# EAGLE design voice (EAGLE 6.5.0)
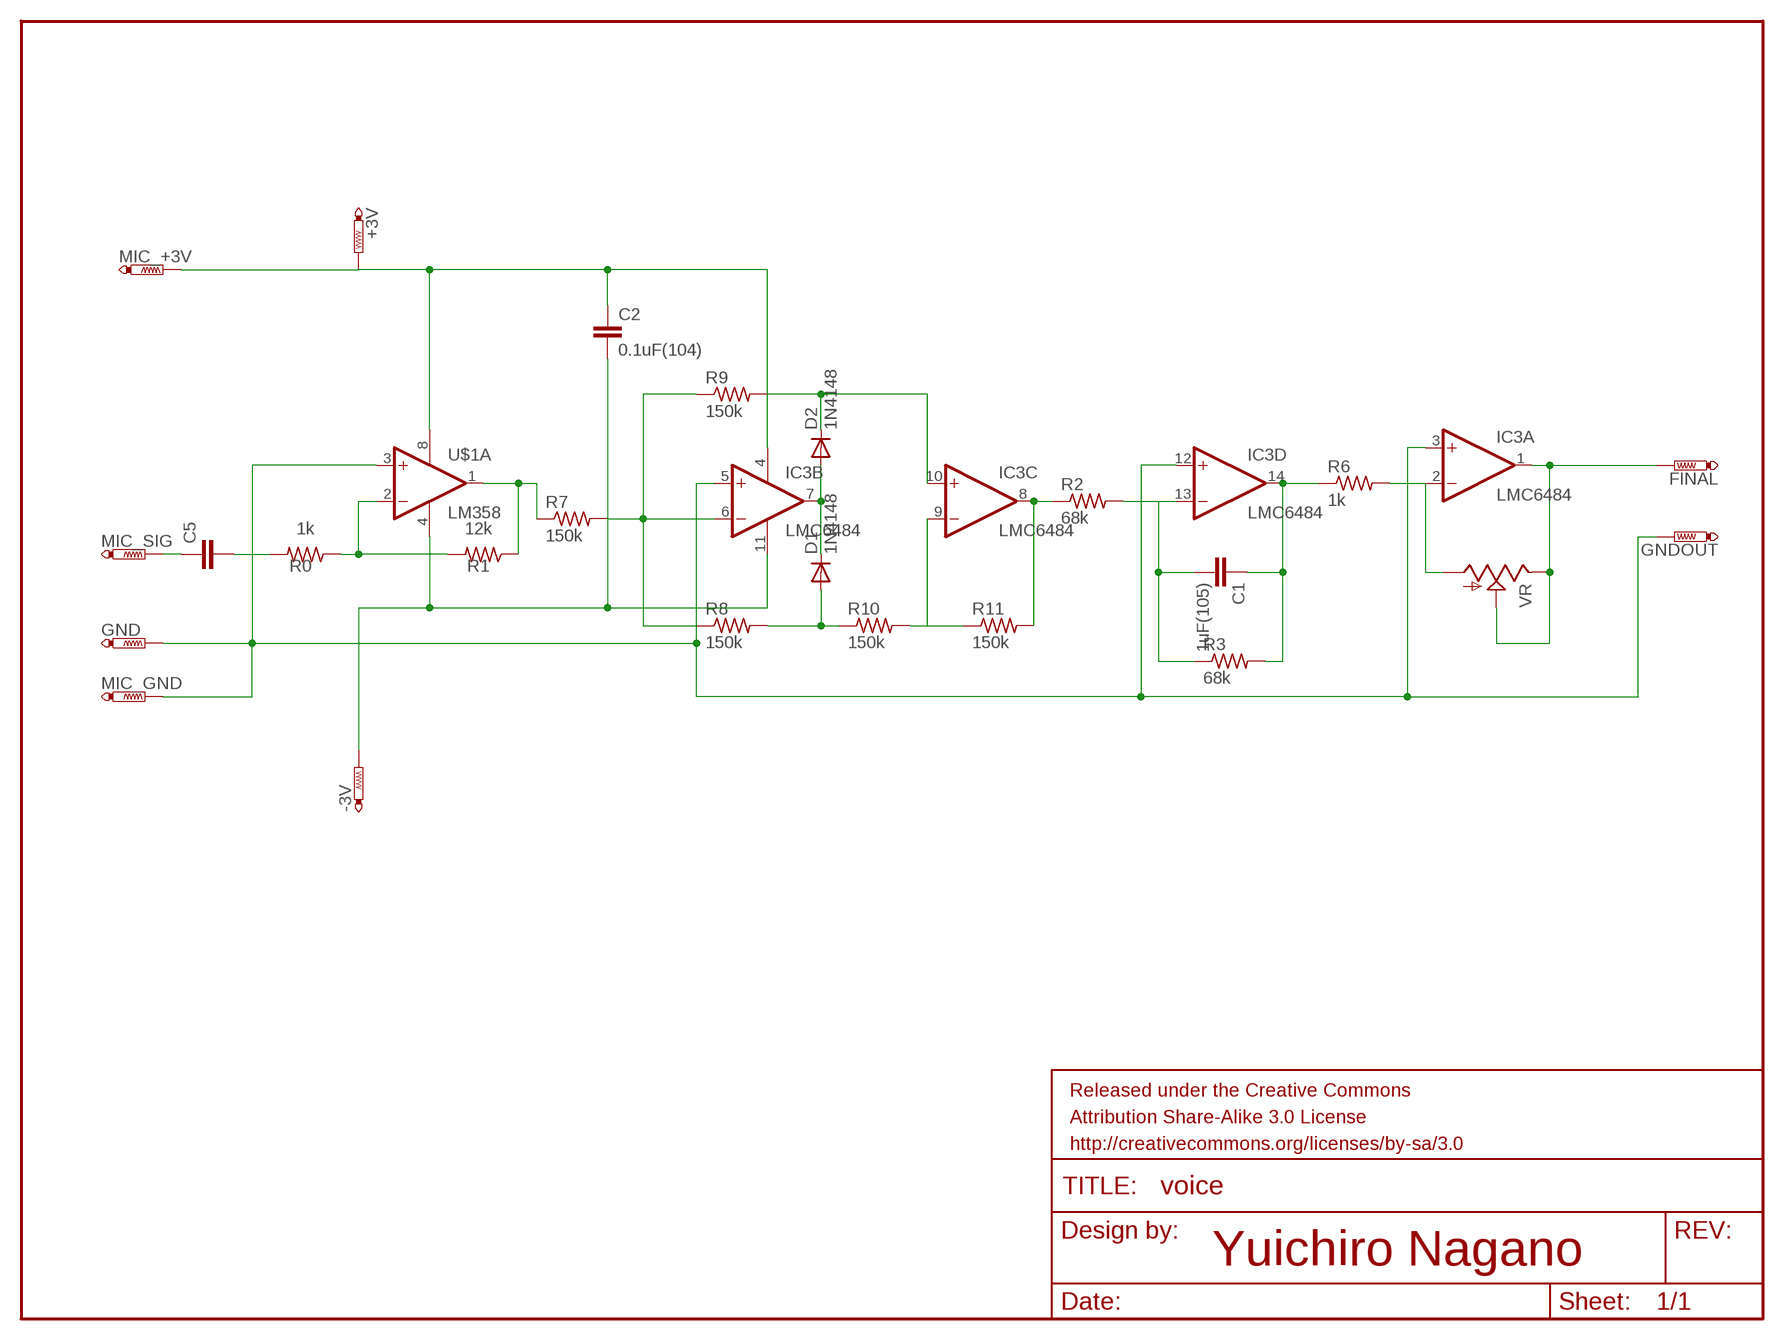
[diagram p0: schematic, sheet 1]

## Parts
+3V  PTR1PAD1-13Y  [P1-13Y]
-3V  PTR1PAD1-13Y  [P1-13Y]
C1  1uF(105)  C2,5-3  [C2.5-3]
C2  0.1uF(104)  C2,5-3  [C2.5-3]
C5  C5/5  [C5B5]
D1  1N4148  1N4148DO35-7  [DO35-7]
D2  1N4148  1N4148DO35-7  [DO35-7]
FINAL  PTR1PAD1-13Y  [P1-13Y]
FRAME1  FRAME-LETTER  [CREATIVE_COMMONS]
GND  PTR1PAD1-13Y  [P1-13Y]
GNDOUT  PTR1PAD1-13Y  [P1-13Y]
IC3  LMC6484  LM324N  [DIL14]
MIC_+3V  PTR1PAD1-13Y  [P1-13Y]
MIC_GND  PTR1PAD1-13Y  [P1-13Y]
MIC_SIG  PTR1PAD1-13Y  [P1-13Y]
R0  1k  R-US_0204/2V  [0204V]
R1  12k  R-US_0204/2V  [0204V]
R2  68k  R-US_0204/2V  [0204V]
R3  68k  R-US_0204/2V  [0204V]
R6  1k  R-US_0204/2V  [0204V]
R7  150k  R-US_0204/2V  [0204V]
R8  150k  R-US_0204/2V  [0204V]
R9  150k  R-US_0204/2V  [0204V]
R10  150k  R-US_0204/2V  [0204V]
R11  150k  R-US_0204/2V  [0204V]
U$1  LM358  [DIL8]
VR  TRIM_US-B25P  [B25P]

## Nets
N$1: IC3.9(C:-IN) R10.2 R11.1
N$2: D1.C D2.A IC3.7(B:OUT)
N$3: -3V.TP C2.2 IC3.11(P:V-) U$1.4(P:V-)
N$4: R1.1 R7.1 U$1.1(A:OUT)
N$5: R0.1 R1.2 U$1.2(A:-IN)
N$6: C5.1 MIC_SIG.TP
N$7: D1.A R8.2 R10.1
N$8: +3V.TP C2.1 IC3.4(P:V+) MIC_+3V.TP U$1.8(P:V+)
N$9: C5.2 R0.2
N$10: IC3.8(C:OUT) R2.1 R11.2
N$12: GND.TP GNDOUT.TP IC3.3(A:+IN) IC3.5(B:+IN) IC3.12(D:+IN) MIC_GND.TP U$1.3(A:+IN)
N$15: IC3.6(B:-IN) R7.2 R8.1 R9.1
N$16: D2.C IC3.10(C:+IN) R9.2
N$17: C1.2 IC3.13(D:-IN) R2.2 R3.1
N$18: C1.1 IC3.14(D:OUT) R3.2 R6.1
N$19: IC3.2(A:-IN) R6.2 VR.A
N$21: FINAL.TP IC3.1(A:OUT) VR.E VR.S
Unconnected: U$1.5(B:+IN) U$1.6(B:-IN) U$1.7(B:OUT)

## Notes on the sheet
- Yuichiro Nagano

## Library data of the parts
+3V -3V FINAL GND GNDOUT MIC_+3V MIC_GND MIC_SIG = testpad:PTR1: TEST PIN
C1 C2 C5 = capacitor-wima:C: CAPACITOR
D1 D2 = diode:1N4148: DIODE
FRAME1 = SparkFun-Aesthetics:FRAME-LETTER: Schematic Frame
IC3 = linear:LM324: OP AMP
R0 R1-R3 R6-R11 = resistor:R-US_: RESISTOR, American symbol
U$1 = atari:LM358: Dual General Purpose, Rail-to-Rail Output Operational Amplifier
VR = pot:TRIM_US-: POTENTIOMETER

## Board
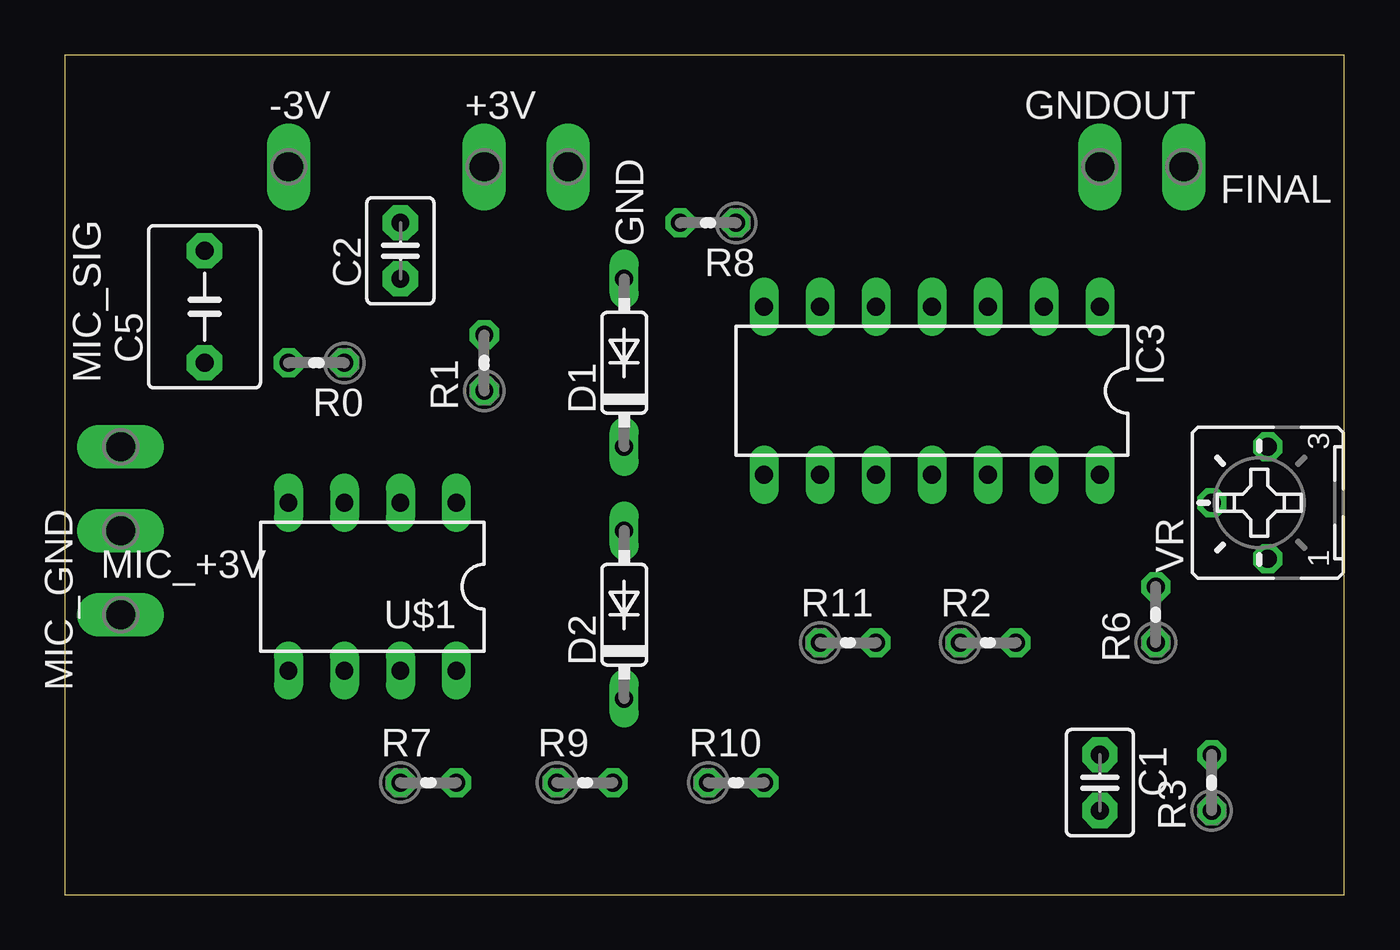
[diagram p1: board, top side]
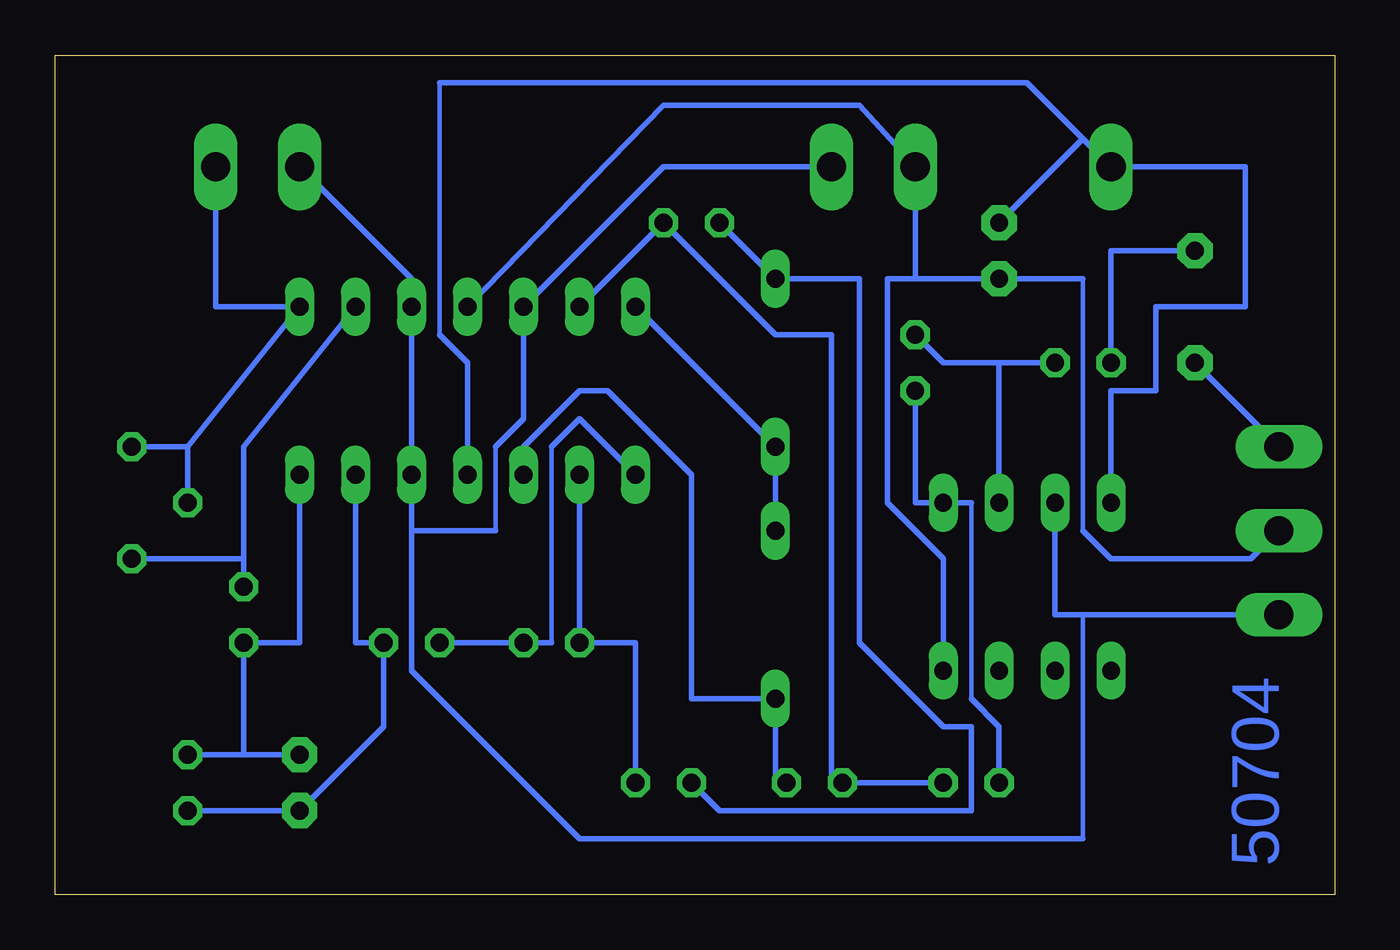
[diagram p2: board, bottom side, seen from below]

Size 58.09 x 38.09 mm. Coordinates in mm from the lower left corner, seen from the top.
Outline: 0,0 58.09,0 58.09,38.09 0,38.09 0,0
Copper layers (1*16): Top 0.035mm / dielectric 1.5mm / Bottom 0.035mm
Design rules "default": minimum track width 10mil, minimum drill 24mil, track to track 8mil, track to pad 8mil, pad to pad 8mil, via to via 8mil, smd to smd 8mil, copper to edge 40mil, drill to drill 8mil, minimum pad ring 10mil, minimum via ring 8mil, stop-mask expansion 4mil, vias tented up to drill 0mil, thermal gap 10mil

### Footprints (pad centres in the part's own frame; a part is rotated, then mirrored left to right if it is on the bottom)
P1-13Y = drill 1.321 pad 1.905 long: TP 0,0
C2.5-3 = drill 0.813 pad 1.6 octagon: 1 -1.27,0; 2 1.27,0
C5B5 = drill 0.813 pad 1.6 octagon: 1 -2.54,0; 2 2.54,0
DO35-7 = drill 0.813 long: A 3.81,0; C -3.81,0
DIL14 = drill 0.813 long: 1 -7.62,-3.81; 2 -5.08,-3.81; 3 -2.54,-3.81; 4 0,-3.81; 5 2.54,-3.81; 6 5.08,-3.81; 7 7.62,-3.81; 8 7.62,3.81; 9 5.08,3.81; 10 2.54,3.81; 11 0,3.81; 12 -2.54,3.81; 13 -5.08,3.81; 14 -7.62,3.81
0204V = drill 0.813 octagon: 1 -1.27,0; 2 1.27,0
DIL8 = drill 0.813 long: 1 -3.81,-3.81; 2 -1.27,-3.81; 3 1.27,-3.81; 4 3.81,-3.81; 5 3.81,3.81; 6 1.27,3.81; 7 -1.27,3.81; 8 -3.81,3.81
B25P = drill 0.813 octagon: A -2.54,0; E 2.54,0; S 0,2.54

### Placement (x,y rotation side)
+3V  19.05,33.02 0 top
-3V  10.16,33.02 0 top
C1  46.99,5.08 270 top
C2  15.24,29.21 90 top
C5  6.35,26.67 90 top
D1  25.4,24.13 90 top
D2  25.4,12.7 90 top
FINAL  50.8,33.02 0 top
FRAME1  not placed on the board
GND  22.86,33.02 180 top
GNDOUT  46.99,33.02 0 top
IC3  39.37,22.86 180 top
MIC_+3V  2.54,16.51 90 top
MIC_GND  2.54,12.7 90 top
MIC_SIG  2.54,20.32 90 top
R0  11.43,24.13 180 top
R1  19.05,24.13 90 top
R2  41.91,11.43 0 top
R3  52.07,5.08 90 top
R6  49.53,12.7 90 top
R7  16.51,5.08 0 top
R8  29.21,30.48 180 top
R9  23.62,5.08 0 top
R10  30.48,5.08 0 top
R11  35.56,11.43 0 top
U$1  13.97,13.97 180 top
VR  54.61,17.78 90 top

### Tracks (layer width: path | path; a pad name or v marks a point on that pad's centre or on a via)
N$1
  Bottom 0.254: R10.2 31.75,11.43 R11.1 IC3.9
N$2
  Bottom 0.254: D2.A D1.C IC3.7
N$3
  Bottom 0.203: 40.64,36.83 40.64,25.4
  Bottom 0.254: U$1.4 10.16,22.86 8.13,22.86 8.13,26.67 4.06,26.67 4.06,33.02 -3V.TP 11.43,34.29 | IC3.11 39.37,24.13 40.64,25.4 | 40.64,36.83 13.97,36.83 11.43,34.29 | 11.43,34.29 C2.2
N$4
  Bottom 0.203: 16.51,17.78 16.51,8.89
  Bottom 0.254: R7.1 15.24,7.62 16.51,8.89 | 16.51,17.78 U$1.1 19.05,17.78 R1.1
N$5
  Bottom 0.254: 15.24,24.13 U$1.2 | R0.1 15.24,24.13 | R1.2 17.78,24.13 15.24,24.13
N$6
  Bottom 0.254: MIC_SIG.TP C5.1
N$7
  Bottom 0.254: R8.2 D1.A 21.59,27.94 21.59,11.43 17.78,7.62 16.51,7.62 16.51,3.81 27.94,3.81 R10.1
N$8
  Bottom 0.203: 11.43,27.94 11.43,16.51
  Bottom 0.254: IC3.4 30.48,35.81 21.59,35.81 +3V.TP 19.05,27.94 | U$1.8 17.78,15.24 20.32,17.78 20.32,27.94 19.05,27.94 | 19.05,27.94 C2.1 11.43,27.94 | MIC_+3V.TP 3.81,15.24 10.16,15.24 11.43,16.51
N$9
  Bottom 0.254: R0.2 10.16,29.21 C5.2
N$10
  Bottom 0.203: 35.56,11.43 35.56,20.32
  Bottom 0.254: R2.1 R11.2 35.56,11.43 | IC3.8 34.29,21.59 35.56,20.32
N$12
  Bottom 0.203: 11.43,2.54 11.43,12.7 | 38.1,16.51 38.1,20.32
  Bottom 0.254: GND.TP 30.48,33.02 IC3.5 36.83,21.59 38.1,20.32 | U$1.3 12.7,12.7 11.43,12.7 MIC_GND.TP | GNDOUT.TP 41.91,27.94 IC3.3 IC3.12 41.91,16.51 | 11.43,2.54 34.29,2.54 41.91,10.16 41.91,16.51 | 41.91,16.51 38.1,16.51
N$15
  Bottom 0.254: R7.2 R9.1 22.86,5.08 22.86,25.4 25.4,25.4 R8.1 IC3.6
N$16
  Bottom 0.254: R9.2 25.4,5.08 D2.C 29.21,8.89 29.21,19.05 33.02,22.86 34.29,22.86 36.83,20.32 IC3.10
N$17
  Bottom 0.254: R3.1 C1.2 43.18,7.62 R2.2 44.45,11.43 IC3.13
N$18
  Bottom 0.254: C1.1 49.53,6.35 | 49.53,6.35 R3.2 | 49.53,6.35 R6.1 46.99,11.43 IC3.14
N$19
  Bottom 0.254: 49.53,15.24 R6.2 | VR.A 49.53,15.24 | IC3.2 49.53,20.32 49.53,15.24
N$21
  Bottom 0.254: 52.07,20.32 IC3.1 50.8,26.67 FINAL.TP | VR.E 52.07,20.32 | 52.07,20.32 VR.S

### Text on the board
Bottom: 50704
